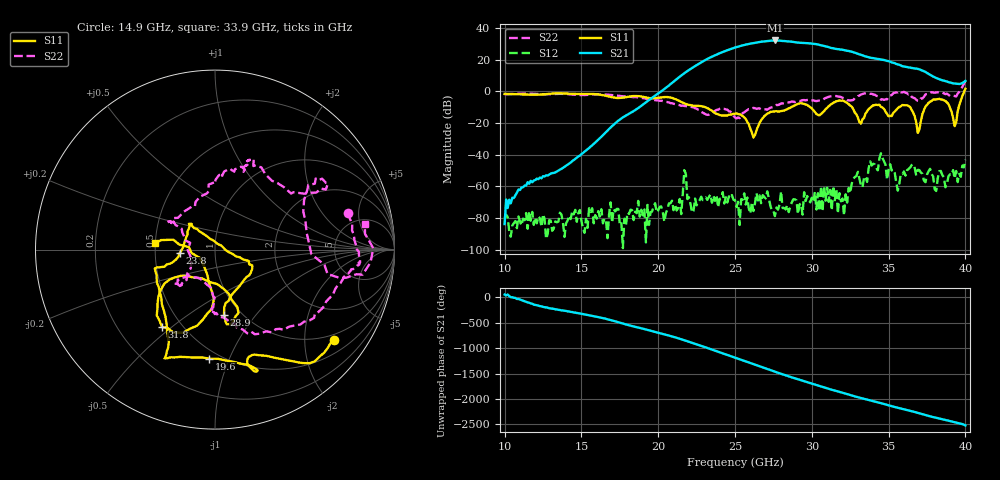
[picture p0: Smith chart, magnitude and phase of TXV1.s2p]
!Keysight Technologies,M9808A,MY58100618,A.14.70.03
!Date: Monday, February 27, 2023 13:37:18
!Correction: S11(C  2-Port  )
!S21(C  2-Port  )
!S12(C  2-Port  )
!S22(C  2-Port  )
!S2P File: Measurements: S11, S21, S12, S22:
# Hz S  RI  R 50
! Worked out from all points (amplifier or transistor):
!   301 points, 10 GHz to 40 GHz, reference 50 ohm
!   highest |S21| = 32.2 dB at 27.6 GHz (marker M1)
!   |S21| within 3 dB of that: 25.54 GHz to 30.58 GHz (5.038 GHz wide, 18 % of centre)
!   unconditionally stable (mu >= 1): start of sweep to 35.66 GHz; 35.75 GHz to 39.62 GHz
!   at 15 GHz: K = 74568.09, MAG = -30.7 dB, |S12| = -81.7 dB
!   at 25 GHz: K = 51.98, MAG = 28.0 dB, |S12| = -68.7 dB
!   at 40 GHz: K = 59.90, MSG = 24.9 dB, |S12| = -43.1 dB
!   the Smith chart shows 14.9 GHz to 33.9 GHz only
!   S11 on the Smith chart (normalised r, x): 14.9 GHz: 0.83, -2.75; 19.6 GHz: 0.44, -0.85; 23.8 GHz: 0.67, -0.03; 28.9 GHz: 0.84, -0.70; 31.8 GHz: 0.39, -0.46; 33.9 GHz: 0.50, +0.04
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1e10  0.7129 0.4426  4.24e-05 4.88e-05  -1.41e-05 -9.35e-05  0.0844 0.8179
1.49e10  0.6637 -0.5037  0.00756 0.00559  -0.000133 -0.000122  0.7433 0.2054
1.5e10  0.6446 -0.5197  0.00889 0.00548  8.18e-05 -8.21e-06  0.7494 0.1768
1.96e10  -0.0322 -0.6074  0.3891 0.4977  0.000109 -0.000117  0.3141 -0.4608
2e10  -0.1946 -0.5976  0.8129 0.2935  -0.000101 -0.000144  0.2218 -0.4718
2.26e10  -0.3361 -0.1056  -5.813 4.381  0.000217 -0.000215  -0.00147 -0.2672
2.38e10  -0.1974 -0.0203  13.95 4.556  -0.000352 0.000407  -0.2011 -0.1678
2.5e10  -0.1407 0.1389  -7.532 -23.29  0.000369 2.08e-06  -0.1325 -0.0731
2.58e10  -0.0649 0.0882  -30.32 7.225  -6.54e-05 -0.000439  -0.2194 0.1368
2.66e10  0.0994 -0.0248  4.734 36.22  -0.00015 -0.000499  -0.2327 0.1756
2.72e10  0.1909 -0.082  37.53 12.84  3.07e-05 0.000434  -0.1085 0.2657
2.76e10  0.1996 -0.1278  37.38 -16.71  -0.000115 1.35e-05  -0.0354 0.3623
2.82e10  0.1231 -0.2182  2.531 -39.27  0.000182 9.88e-05  0.0395 0.4115
2.89e10  0.0504 -0.3623  -32.51 -15.43  -0.000297 -0.000249  0.1582 0.4332
2.94e10  0.0994 -0.402  -32.16 11.76  -0.000125 -2.86e-05  0.1863 0.4991
3e10  0.0925 -0.2784  -6.91 31.95  -0.000208 -0.000389  0.2219 0.4679
3.08e10  -0.1895 -0.1459  24.8 11.7  -0.00101 -0.000127  0.4973 0.3116
3.18e10  -0.2947 -0.4317  10.7 -18.75  0.000352 0.000504  0.5608 0.3959
3.28e10  -0.0242 -0.2133  -14.32 -8.763  -0.00109 -0.00165  0.6095 -0.0843
3.39e10  -0.3358 0.0342  -6.651 9.318  0.00134 0.00439  0.835 0.1433
3.5e10  0.00706 -0.1652  7.309 5.39  -0.0033 0.000809  0.6459 -0.2751
4e10  0.5879 -1.067  2.163 0.0244  0.00475 0.00513  1.106 -1.834
